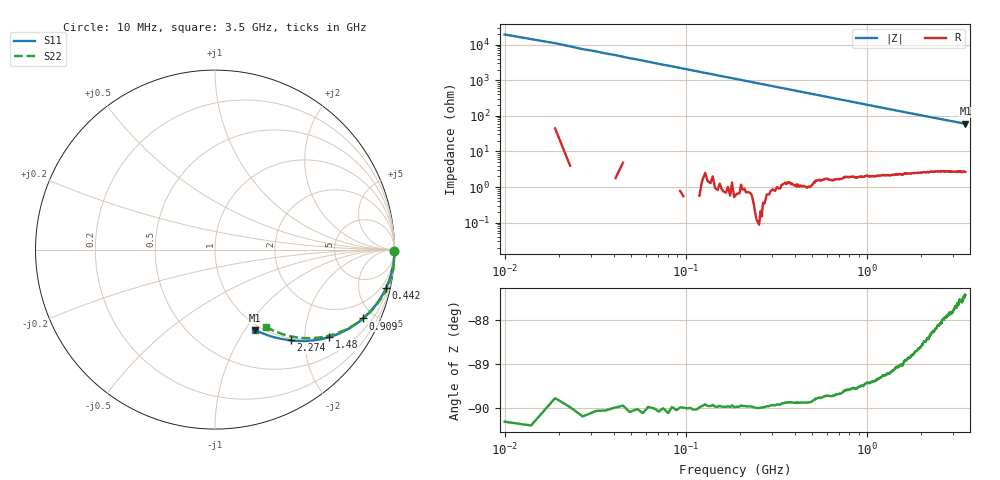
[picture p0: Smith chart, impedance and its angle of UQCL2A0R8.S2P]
! AVX Corporation
! Date:  10/27/06
! Part No:  UQCL2A0R8
! Description:  Ultra Low ESR Microwave capacitors
! Mounting Orientation:  Horizontal
# GHZ S DB R 50
! Freq  |S11|  S11 Ph  |S21|  S21 Ph  |S12|  S12 Ph  |S22|  S22 Ph
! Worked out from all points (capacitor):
!   801 points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, 10 MHz to 3.5 GHz, reference 50 ohm
!   read as one part in series: C = 774 fF near 27 MHz
!   lowest |Z| = 59.9 ohm at 3.5 GHz (marker M1)
!   S11 on the Smith chart (normalised r, x): 10 MHz: open; 442 MHz: 0.97, -8.86; 909 MHz: 0.98, -4.31; 1.48 GHz: 0.97, -2.64; 2.274 GHz: 0.96, -1.72; 3.5 GHz: 0.93, -1.11
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0.01  -0.01 -0.3  -45.73 89.9  -46.26 90.0  -0.01 -0.4
0.019  -0.01 -0.6  -40.84 89.2  -40.82 89.2  -0.01 -0.5
0.036  -0.01 -1.1  -35.10 89.0  -35.08 88.9  -0.01 -1.0
0.049  -0.01 -1.5  -32.42 88.7  -32.37 88.2  -0.01 -1.4
0.062  -0.01 -1.9  -30.38 88.2  -30.35 88.3  -0.01 -1.8
0.075  -0.01 -2.2  -28.73 87.8  -28.68 87.8  -0.01 -2.2
0.097  -0.01 -2.9  -26.54 87.2  -26.49 87.2  -0.01 -2.8
0.123  -0.02 -3.6  -24.47 86.4  -24.42 86.4  -0.01 -3.5
0.171  -0.04 -5.0  -21.63 85.0  -21.58 85.0  -0.01 -4.9
0.254  -0.07 -7.4  -18.24 82.7  -18.19 82.7  -0.02 -7.2
0.328  -0.11 -9.5  -16.05 80.5  -16.01 80.5  -0.06 -9.3
0.442  -0.21 -12.7  -13.56 77.3  -13.52 77.3  -0.16 -12.4
0.595  -0.37 -16.9  -11.14 73.0  -11.10 73.0  -0.32 -16.5
0.747  -0.57 -20.9  -9.36 69.0  -9.32 68.9  -0.52 -20.4
0.909  -0.83 -25.0  -7.93 64.8  -7.89 64.8  -0.77 -24.4
1.175  -1.30 -31.1  -6.19 58.7  -6.15 58.6  -1.25 -30.2
1.48  -1.92 -37.4  -4.84 52.5  -4.79 52.4  -1.86 -36.0
1.755  -2.50 -42.3  -3.98 47.6  -3.94 47.5  -2.44 -40.5
2.274  -3.61 -50.0  -2.93 40.2  -2.89 40.1  -3.52 -47.1
2.34  -3.74 -50.9  -2.83 39.4  -2.79 39.3  -3.65 -47.8
2.92  -4.91 -57.7  -2.19 33.5  -2.15 33.4  -4.77 -53.0
3.5  -6.04 -63.8  -1.80 29.0  -1.77 28.9  -5.79 -56.7
